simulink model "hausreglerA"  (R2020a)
settings: Solver=ode45  StartTime=0.0  StopTime=400  MaxStep=1  RelTol=1e-3  EnableMultiTasking=on
libraries: libregler1B x1

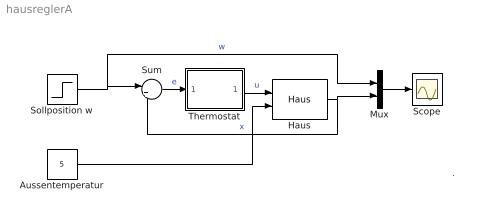
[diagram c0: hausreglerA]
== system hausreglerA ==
  note: .
  Aussentemperatur : Constant  Value=5
  Haus : libregler1B/Haus  C=100000  R=0.001  T0=16
  Mux : Mux  Inputs=2
  Scope : Scope
  Sollposition w : Step  After=20  SampleTime=0
  Sum : Sum  Inputs=|+-  SaturateOnIntegerOverflow=on
  Thermostat : Subsystem  mask{umax=18500}
      mask prompts: umax "Schaltwert"
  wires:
  Thermostat/1(Out1) -> Haus/1  "u"
  Haus/1 -> Sum/2, Mux/2  "x"
  Sollposition w/1 -> Sum/1, Mux/1  "w"
  Sum/1 -> Thermostat/1(In1)  "e"
  Mux/1 -> Scope/1
  Aussentemperatur/1 -> Haus/2

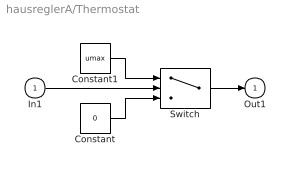
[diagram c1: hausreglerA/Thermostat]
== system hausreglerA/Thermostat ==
  In1 : Inport
  Constant : Constant  Value=0
  Constant1 : Constant  Value=umax
  Switch : Switch  Criteria=u2 > Threshold
  Out1 : Outport  InitialOutput=0
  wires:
  Switch/1 -> Out1/1
  In1/1 -> Switch/2
  Constant/1 -> Switch/3
  Constant1/1 -> Switch/1
